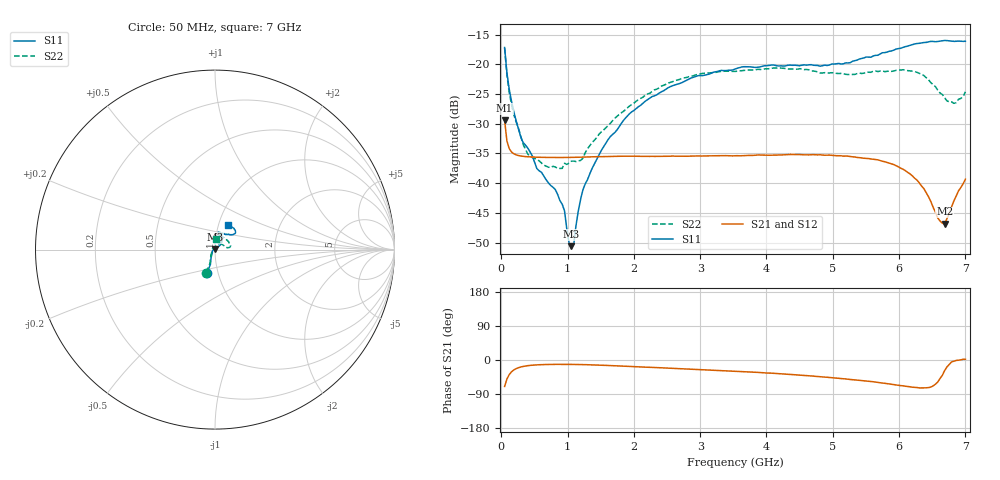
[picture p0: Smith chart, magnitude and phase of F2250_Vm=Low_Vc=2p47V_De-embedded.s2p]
! Integrated Device Technology
! Corporate Headquarters
! 6024 Silver Creek Valley Road
! San Jose, CA 95138  USA
! Phone:  1-408-284-8200
! Toll Free:  1-800-223-1366
! Webpage:  http://www.idt.com/
! Timing and RF Division
! 515 Groton Road, Suite 102
! Westford, MA 01886-6024
! Device:  F2250
! Description: Voltage Variable RF Attenuator
! Frequency:  50.0 -  6000.00 MHz
! Package:  3x3 mm Thin QFN Plastic Package: 16 pin
! Ports:  2 RF, 3 DC
!  Pin  1  = GND
!  Pin  2  = NC
!  Pin  3  = RF1  = Port 1
!  Pin  4  = NC
!  Pin  5  = GND
!  Pin  6  = GND
!  Pin  7  = GND
!  Pin  8  = GND
!  Pin  9  = NC
!  Pin 10  = RF2  = Port 2
!  Pin 11  = NC
!  Pin 12  = GND
!  Pin 13  = GND
!  Pin 14  = VCNTRL
!  Pin 15  = VDD
!  Pin 16  = VMODE
! Vcntrl:  2.470 Volts
! Vmode:  +0.000 Volts
! Vdd:  +3.30  Volts
! Current:  1.175 mA
! Data:  The device was measured on a the F2250 evaluation board which has
!  individual transmission lines to the RF pins.  Data was collected
!  using a calibrated network analyzer.  The evaluation board was
!  de-embedded using a TRL calibration technique.
!  The reference plane is the edge of the package pin.
! Misc:  SN 10
!  Action Tracker AT0258
! Date Measured:  2014-11-26
! Date:  2015-10-15  MJV
! Note:
!  Integrated Device Technology supplies this data as a sample of measured
!  data at the package pin for this product.  Your particular data for this
!  product may vary.
!  Data was taken at 25 degrees C.
!  Integrated Device Technology reserves the right to change this data at anytime.
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# GHz S dB R 50
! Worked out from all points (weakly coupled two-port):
!   201 points, 50 MHz to 7 GHz, reference 50 ohm
!   highest |S21| = -29.41 dB at 50 MHz (marker M1); lowest = -46.8 dB at 6.687 GHz (marker M2)
!   lowest |S11| = -50.6 dB at 1.058 GHz (marker M3), VSWR 1.01, Z = 49.8 + j0.247 ohm
!   |S11| at or under -10 dB: start of sweep to end of sweep
!   |S22| runs from -37.5 to -17.3 dB; largest |S21 - S12| = 5.5e-05
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0.05  -17.18 -108.6  -29.41 -69.8  -29.41 -69.8  -17.28 -111.0
0.08475  -21.45 -107.4  -32.92 -50.4  -32.92 -50.4  -21.75 -110.2
0.15425  -26.23 -116.6  -34.76 -31.2  -34.75 -31.1  -26.82 -122.3
0.29325  -32.20 -127.8  -35.43 -18.5  -35.43 -18.5  -32.10 -137.6
0.3975  -34.08 -141.9  -35.56 -15.0  -35.56 -15.0  -35.05 -160.5
0.91875  -43.55 157.8  -35.69 -11.5  -35.68 -11.5  -37.52 133.5
0.9535  -44.65 170.0  -35.68 -11.5  -35.68 -11.5  -36.65 131.2
1.023  -50.09 144.2  -35.67 -11.6  -35.67 -11.6  -36.62 115.9
1.05775  -50.61 122.9  -35.67 -11.6  -35.67 -11.6  -36.29 110.7
1.0925  -50.34 90.1  -35.66 -11.7  -35.65 -11.7  -36.29 106.2
1.162  -44.65 56.9  -35.64 -11.9  -35.64 -11.9  -36.24 95.5
1.2315  -41.11 44.3  -35.61 -12.1  -35.61 -12.1  -35.80 85.9
1.6485  -32.11 42.0  -35.52 -14.6  -35.52 -14.6  -29.89 64.5
1.96125  -28.05 42.2  -35.46 -17.2  -35.46 -17.2  -26.81 56.9
2.37825  -24.87 47.3  -35.48 -20.3  -35.47 -20.3  -23.99 56.8
3.525  -20.80 72.4  -35.41 -29.5  -35.41 -29.5  -21.19 74.8
4.7065  -20.16 72.3  -35.21 -42.5  -35.20 -42.5  -21.14 72.3
5.85325  -17.81 40.5  -36.64 -63.2  -36.64 -63.3  -21.13 23.0
6.27025  -16.50 40.1  -39.49 -72.6  -39.50 -72.6  -21.36 9.7
6.68725  -15.99 48.8  -46.84 -27.8  -46.81 -27.4  -25.64 28.5
6.861  -16.13 55.1  -42.17 -1.2  -42.14 -1.2  -26.46 57.9
7  -16.12 63.2  -39.34 1.9  -39.31 1.8  -24.63 83.1
